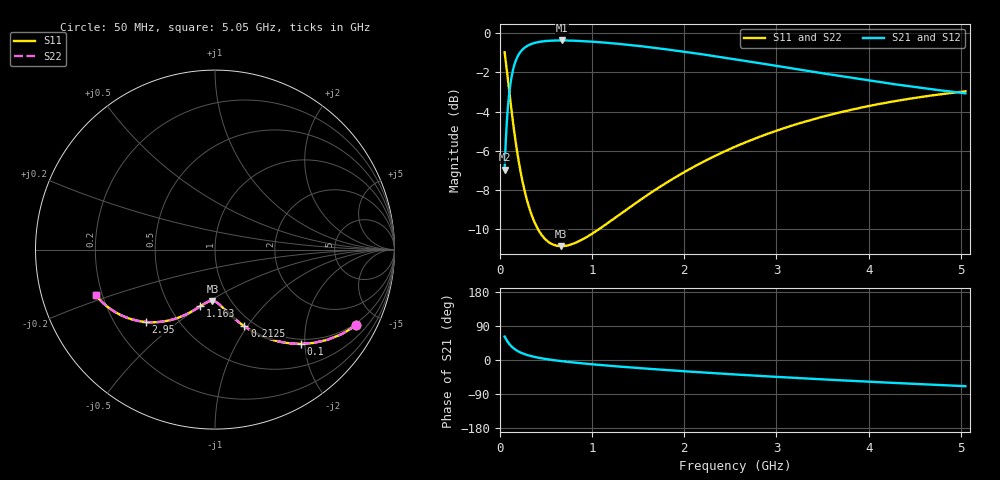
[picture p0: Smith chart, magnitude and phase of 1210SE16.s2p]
! AVX Thin Film Operation		Date: August 2001
! Description: Accu-P® Series, Thin Film, SMD, RF Capacitor
! Part Number: 12101J16FBT
! 50 MHz  -  5.05 GHz
! Serial Measurements
# mhz S db R 50
!	S11		S21		S12		S22
!	dB	Phase	dB	Phase	dB	Phase	dB	Phase
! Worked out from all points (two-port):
!   401 points, 50 MHz to 5.05 GHz, reference 50 ohm
!   highest |S21| = -0.37 dB at 675 MHz (marker M1); lowest = -7.0 dB at 50 MHz (marker M2)
!   |S21| within 3 dB of the highest: 93.79 MHz to end of sweep
!   lowest |S11| = -10.9 dB at 662.5 MHz (marker M3), VSWR 1.80, Z = 41.3 - j25.7 ohm
!   |S11| at or under -10 dB: 411.9 MHz to 1.074 GHz (662.4 MHz wide, 89.1 % of centre)
!   |S22| runs from -10.9 to -1.0 dB; largest |S21 - S12| = 0
!   S11 on the Smith chart (normalised r, x): 50 MHz: 0.90, -3.79; 100 MHz: 0.90, -1.92; 212.5 MHz: 0.90, -0.97; 1.163 GHz: 0.70, -0.50; 2.95 GHz: 0.33, -0.39; 5.05 GHz: 0.17, -0.18
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50  -0.97 -28.1  -6.97 61.9  -6.97 61.9  -0.98 -28.1
75  -1.93 -39.0  -4.46 51.0  -4.46 51.0  -1.93 -39.0
100  -2.95 -47.6  -3.07 42.4  -3.07 42.4  -2.95 -47.6
125  -3.95 -54.3  -2.24 35.7  -2.24 35.7  -3.95 -54.3
150  -4.88 -59.6  -1.71 30.3  -1.71 30.3  -4.88 -59.6
175  -5.71 -64.0  -1.36 26.0  -1.36 26.0  -5.71 -64.0
212.5  -6.80 -69.1  -1.02 20.9  -1.02 20.9  -6.80 -69.1
250  -7.70 -73.0  -0.81 16.9  -0.81 16.9  -7.70 -73.0
287.5  -8.43 -76.2  -0.68 13.7  -0.68 13.7  -8.43 -76.2
400  -9.90 -83.1  -0.47 6.8  -0.47 6.8  -9.90 -83.1
512.5  -10.60 -87.9  -0.40 2.0  -0.40 2.0  -10.60 -87.9
662.5  -10.87 -92.8  -0.37 -2.9  -0.37 -2.9  -10.87 -92.8
675  -10.87 -93.2  -0.37 -3.3  -0.37 -3.3  -10.87 -93.2
887.5  -10.54 -98.7  -0.40 -8.7  -0.40 -8.7  -10.54 -98.7
1162.5  -9.71 -104.7  -0.49 -14.7  -0.49 -14.7  -9.71 -104.7
1725  -7.87 -115.1  -0.78 -25.1  -0.78 -25.1  -7.87 -115.1
2125  -6.76 -121.7  -1.03 -31.7  -1.03 -31.7  -6.76 -121.7
2550  -5.79 -128.1  -1.33 -38.2  -1.33 -38.2  -5.79 -128.1
2950  -5.06 -133.8  -1.63 -43.8  -1.63 -43.8  -5.06 -133.8
3387.5  -4.41 -139.6  -1.96 -49.7  -1.96 -49.7  -4.41 -139.6
4225  -3.52 -149.8  -2.57 -59.9  -2.57 -59.9  -3.52 -149.8
5050  -2.97 -159.0  -3.07 -69.1  -3.07 -69.1  -2.97 -159.0
